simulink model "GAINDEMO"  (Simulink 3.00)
settings: Solver=ode45  SolverMode=SingleTasking  StartTime=0  StopTime=30  MaxStep=1  RelTol=1e-3  AbsTol=1e-3

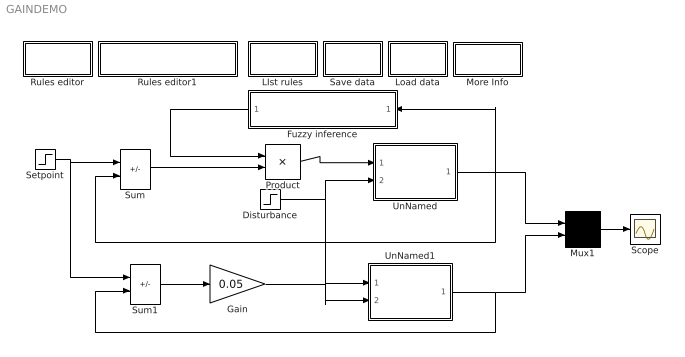
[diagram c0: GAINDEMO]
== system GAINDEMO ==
  Disturbance : Step  Time=2  Before=0  After=0  SampleTime=0
  Fuzzy inference : Subsystem  Orientation=left  mask(Fuzzy inference block){}
      mask help: MIN-MAX inference with fuzzy means defuzzification
      mask init:
      | rls = @1; mfs = @2; def = @3;
  Gain : Gain  Gain=0.05  SaturateOnIntegerOverflow=on
  LIst rules : Subsystem
  Load data : Subsystem
  More Info : Subsystem
  Mux1 : Mux  Inputs=2
  Product : Product  Inputs=2  SaturateOnIntegerOverflow=on
  Rules editor : Subsystem
  Rules editor1 : Subsystem
  Save data : Subsystem
  Scope : Scope
  Setpoint : Step  Time=1  Before=2  After=1  SampleTime=0
  Sum : Sum  Inputs=+-  SaturateOnIntegerOverflow=on
  Sum1 : Sum  Inputs=+-  SaturateOnIntegerOverflow=on
  UnNamed : Subsystem
      mask help: Non-linear 3-rd order process
      mask init:
      | ic = @1;
  UnNamed1 : Subsystem
      mask help: Non-linear 3-rd order process
      mask init:
      | ic = @1;
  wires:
  Mux1/1 -> Scope/1
  Fuzzy inference/1(Out1) -> Product/1
  UnNamed/1(out_1) -> Fuzzy inference/1(In1), Sum/2, Mux1/1
  Sum/1 -> Product/2
  Product/1 -> UnNamed/1(in_1)
  Sum1/1 -> Gain/1
  UnNamed1/1(out_1) -> Mux1/2, Sum1/2
  Gain/1 -> UnNamed1/1(in_1)
  Setpoint/1 -> Sum1/1, Sum/1
  Disturbance/1 -> UnNamed1/2(in_2), UnNamed/2(in_2)

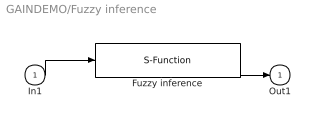
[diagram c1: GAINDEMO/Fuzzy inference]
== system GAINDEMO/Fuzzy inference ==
  In1 : Inport  Port=1  PortWidth=-1  SampleTime=-1  DataType=auto
  Fuzzy inference : S-Function  FunctionName=sfuninf  Parameters=rls, mfs, def  PortCounts=[]  SFunctionModules=''
  Out1 : Outport  Port=1
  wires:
  In1/1 -> Fuzzy inference/1
  Fuzzy inference/1 -> Out1/1

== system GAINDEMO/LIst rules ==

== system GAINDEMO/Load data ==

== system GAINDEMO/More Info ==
  note: To strart click on "Compile rule-base" first. On other systems than MS-Windows, you may want to change the "Edit rules" icon in order to set your preferred text editor.
  note: This demonstration compares a proportional controller vers. fuzzy gain-scheduling control on a nonlinear third-order plant.

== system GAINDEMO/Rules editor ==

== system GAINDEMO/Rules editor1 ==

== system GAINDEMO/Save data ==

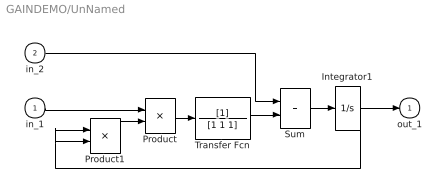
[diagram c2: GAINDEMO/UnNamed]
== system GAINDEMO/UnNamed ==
  in_1 : Inport  Port=1  PortWidth=-1  SampleTime=-1  DataType=auto
  in_2 : Inport  Port=2  PortWidth=-1  SampleTime=-1  DataType=auto
  Integrator1 : Integrator  ExternalReset=none  InitialConditionSource=internal  InitialCondition=ic  LimitOutput=off  UpperSaturationLimit=inf  LowerSaturationLimit=-inf  ShowSaturationPort=off  ShowStatePort=off  AbsoluteTolerance=auto
  Product : Product  Inputs=2  SaturateOnIntegerOverflow=on
  Product1 : Product  Inputs=2  SaturateOnIntegerOverflow=on
  Sum : Sum  Inputs=++  SaturateOnIntegerOverflow=on
  Transfer Fcn : TransferFcn  Numerator=[1]  Denominator=[1 1 1]
  out_1 : Outport  Port=1
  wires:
  Integrator1/1 -> out_1/1, Product1/1, Product1/2
  Sum/1 -> Integrator1/1
  Transfer Fcn/1 -> Sum/2
  in_1/1 -> Product/1
  Product/1 -> Transfer Fcn/1
  Product1/1 -> Product/2
  in_2/1 -> Sum/1

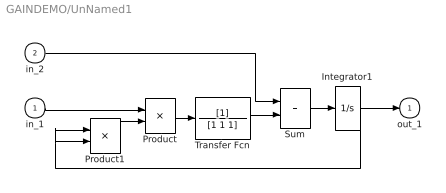
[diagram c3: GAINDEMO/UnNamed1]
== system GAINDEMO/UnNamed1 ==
  in_1 : Inport  Port=1  PortWidth=-1  SampleTime=-1  DataType=auto
  in_2 : Inport  Port=2  PortWidth=-1  SampleTime=-1  DataType=auto
  Integrator1 : Integrator  ExternalReset=none  InitialConditionSource=internal  InitialCondition=ic  LimitOutput=off  UpperSaturationLimit=inf  LowerSaturationLimit=-inf  ShowSaturationPort=off  ShowStatePort=off  AbsoluteTolerance=auto
  Product : Product  Inputs=2  SaturateOnIntegerOverflow=on
  Product1 : Product  Inputs=2  SaturateOnIntegerOverflow=on
  Sum : Sum  Inputs=++  SaturateOnIntegerOverflow=on
  Transfer Fcn : TransferFcn  Numerator=[1]  Denominator=[1 1 1]
  out_1 : Outport  Port=1
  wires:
  Integrator1/1 -> out_1/1, Product1/1, Product1/2
  Sum/1 -> Integrator1/1
  Transfer Fcn/1 -> Sum/2
  in_1/1 -> Product/1
  Product/1 -> Transfer Fcn/1
  Product1/1 -> Product/2
  in_2/1 -> Sum/1
